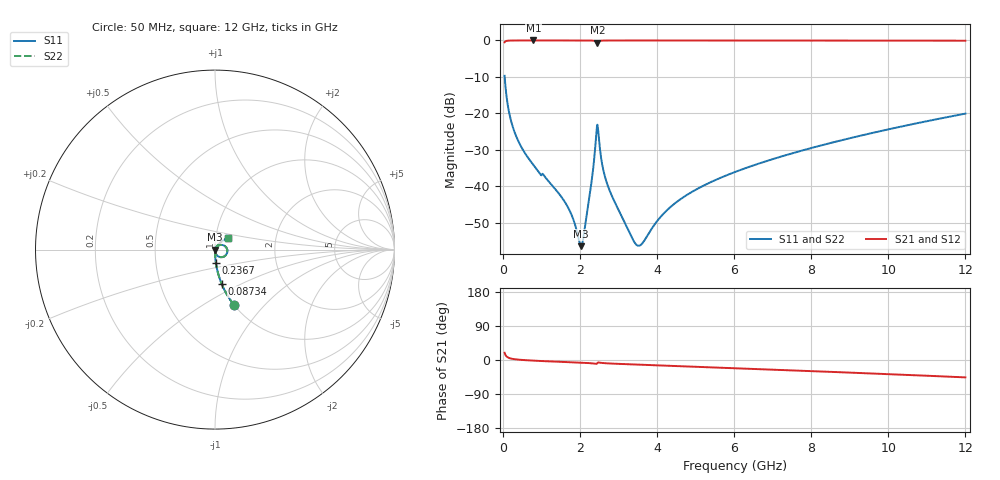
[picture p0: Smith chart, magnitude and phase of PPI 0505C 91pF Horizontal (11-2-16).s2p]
# MHz S MA R 50
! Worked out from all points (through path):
!   1601 points, 50 MHz to 12 GHz, reference 50 ohm
!   highest |S21| = -0.01 dB at 796.9 MHz (marker M1); lowest = -0.6 dB at 2.455 GHz (marker M2)
!   group delay of S21, straight-line fit = 11 ps
!   lowest |S11| = -56.3 dB at 2.037 GHz (marker M3), VSWR 1.00, Z = 50.1 - j0.0292 ohm
!   |S11| at or under -10 dB: 52.14 MHz to end of sweep
!   |S22| runs from -56.3 to -9.7 dB; largest |S21 - S12| = 0
!   S11 on the Smith chart (normalised r, x): 50 MHz: 1.00, -0.69; 87.34 MHz: 1.00, -0.40; 236.7 MHz: 1.00, -0.15; 12 GHz: 1.15, +0.16
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50  0.3279 -71.0  0.9445 19.0  0.9445 19.0  0.3279 -71.0
87.34375  0.1947 -79.0  0.9805 10.9  0.9805 10.9  0.1947 -79.0
236.7188  0.07257 -86.3  0.9969 3.3  0.9969 3.3  0.07257 -86.3
453.3125  0.03717 -88.5  0.9987 0.5  0.9987 0.5  0.03717 -88.5
796.875  0.01973 -89.4  0.999 -1.7  0.999 -1.7  0.01973 -89.4
1625.906  0.005976 -84.4  0.9987 -5.3  0.9987 -5.3  0.005976 -84.4
2036.688  0.001523 -11.0  0.9983 -7.1  0.9983 -7.1  0.001523 -11.0
2044.156  0.001536 -5.5  0.9983 -7.1  0.9983 -7.1  0.001536 -5.5
2141.25  0.002996 44.3  0.998 -7.6  0.998 -7.6  0.002996 44.3
2313.031  0.01255 60.0  0.9952 -8.7  0.9952 -8.7  0.01255 60.0
2417.594  0.04581 35.0  0.9671 -10.3  0.9671 -10.3  0.04581 35.0
2454.938  0.07026 -14.1  0.9299 -8.1  0.9299 -8.1  0.07026 -14.1
2611.781  0.01663 -84.1  0.9956 -8.2  0.9956 -8.2  0.01663 -84.1
2723.812  0.01033 -86.0  0.9975 -8.9  0.9975 -8.9  0.01033 -86.0
3425.875  0.001694 -36.7  0.9982 -11.9  0.9982 -11.9  0.001694 -36.7
3605.125  0.001628 5.5  0.9982 -12.6  0.9982 -12.6  0.001628 5.5
4038.312  0.003531 48.8  0.9981 -14.2  0.9981 -14.2  0.003531 48.8
4800.125  0.007796 60.2  0.9979 -17.1  0.9979 -17.1  0.007796 60.2
6025  0.01579 61.3  0.9976 -21.7  0.9976 -21.7  0.01579 61.3
8019.156  0.0338 56.7  0.9966 -29.4  0.9966 -29.4  0.0338 56.7
10013.31  0.06077 50.0  0.9948 -37.4  0.9948 -37.4  0.06077 50.0
12000  0.09951 42.3  0.9911 -45.9  0.9911 -45.9  0.09951 42.3
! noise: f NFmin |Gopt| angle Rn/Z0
50  0.0003706  0.8582  0.4081  0.000559
1372  0.003804  0.6613  4.838  0.002144
2701  0.008255  0.6886  9.461  0.00512
4031  0.008249  0.57  13.97  0.00342
5360  0.01017  0.5464  18.42  0.003898
6682  0.01207  0.5321  22.75  0.004388
8012  0.01397  0.5234  26.99  0.004889
9341  0.0159  0.5191  31.09  0.005411
1.067e+04  0.01789  0.5186  35.06  0.005968
1.2e+04  0.01997  0.5213  38.89  0.006576
